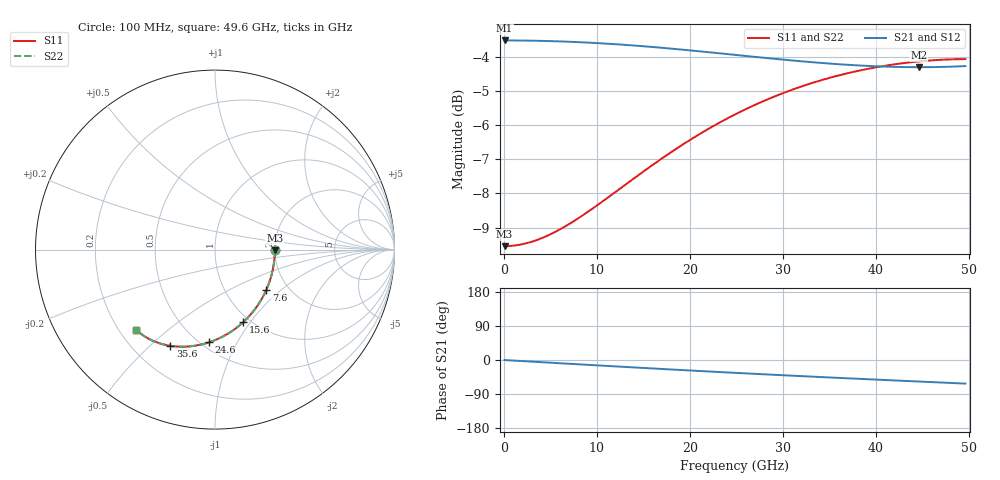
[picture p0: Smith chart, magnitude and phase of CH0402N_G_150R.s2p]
# GHz S RI R 150
! S-Parameters data
! Freq  reS11  imS11  reS21  imS21  reS12  imS12  reS22  imS22
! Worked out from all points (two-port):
!   100 points, 100 MHz to 49.6 GHz, reference 150 ohm
!   highest |S21| = -3.52 dB at 100 MHz (marker M1); lowest = -4.3 dB at 44.6 GHz (marker M2)
!   |S21| within 3 dB of the highest: start of sweep to end of sweep
!   lowest |S11| = -9.5 dB at 100 MHz (marker M3), VSWR 2.00, Z = 300 - j2.07 ohm
!   |S11| at or under -10 dB: nowhere
!   |S22| runs from -9.5 to -4.1 dB; largest |S21 - S12| = 0
!   S11 on the Smith chart (normalised r, x): 100 MHz: 2.00, -0.01; 7.6 GHz: 1.55, -0.80; 15.6 GHz: 0.92, -0.92; 24.6 GHz: 0.55, -0.77; 35.6 GHz: 0.35, -0.58; 49.6 GHz: 0.27, -0.39
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0.1  0.3333 -0.00306  0.6667 -0.00165  0.6667 -0.00165  0.3333 -0.00306
1.6  0.3312 -0.0489  0.666 -0.0263  0.666 -0.0263  0.3312 -0.0489
3.6  0.3224 -0.1093  0.6633 -0.0591  0.6633 -0.0591  0.3224 -0.1093
5.6  0.3073 -0.1678  0.6585 -0.0916  0.6585 -0.0916  0.3073 -0.1678
7.6  0.2862 -0.2236  0.6517 -0.1235  0.6517 -0.1235  0.2862 -0.2236
8.6  0.2736 -0.2501  0.6475 -0.1392  0.6475 -0.1392  0.2736 -0.2501
12.1  0.2202 -0.335  0.6294 -0.1923  0.6294 -0.1923  0.2202 -0.335
15.6  0.1557 -0.4055  0.6062 -0.2422  0.6062 -0.2422  0.1557 -0.4055
16.6  0.1359 -0.4228  0.5988 -0.2557  0.5988 -0.2557  0.1359 -0.4228
18.6  0.0948 -0.4536  0.5829 -0.2817  0.5829 -0.2817  0.0948 -0.4536
20.6  0.0526 -0.4793  0.566 -0.3064  0.566 -0.3064  0.0526 -0.4793
22.6  0.00998 -0.5002  0.5482 -0.3295  0.5482 -0.3295  0.00998 -0.5002
24.6  -0.0326 -0.5164  0.5297 -0.3513  0.5297 -0.3513  -0.0326 -0.5164
25.1  -0.0432 -0.5198  0.5249 -0.3565  0.5249 -0.3565  -0.0432 -0.5198
27.1  -0.085 -0.5306  0.5058 -0.3766  0.5058 -0.3766  -0.085 -0.5306
29.1  -0.1258 -0.5375  0.4863 -0.3953  0.4863 -0.3953  -0.1258 -0.5375
33.1  -0.2032 -0.5405  0.4468 -0.4294  0.4468 -0.4294  -0.2032 -0.5405
35.6  -0.248 -0.5361  0.422 -0.4486  0.422 -0.4486  -0.248 -0.5361
38.6  -0.2978 -0.5253  0.3924 -0.4702  0.3924 -0.4702  -0.2978 -0.5253
41.6  -0.3429 -0.5094  0.3629 -0.4904  0.3629 -0.4904  -0.3429 -0.5094
44.6  -0.3832 -0.489  0.3336 -0.5098  0.3336 -0.5098  -0.3832 -0.489
49.6  -0.4389 -0.4465  0.2843 -0.5415  0.2843 -0.5415  -0.4389 -0.4465
